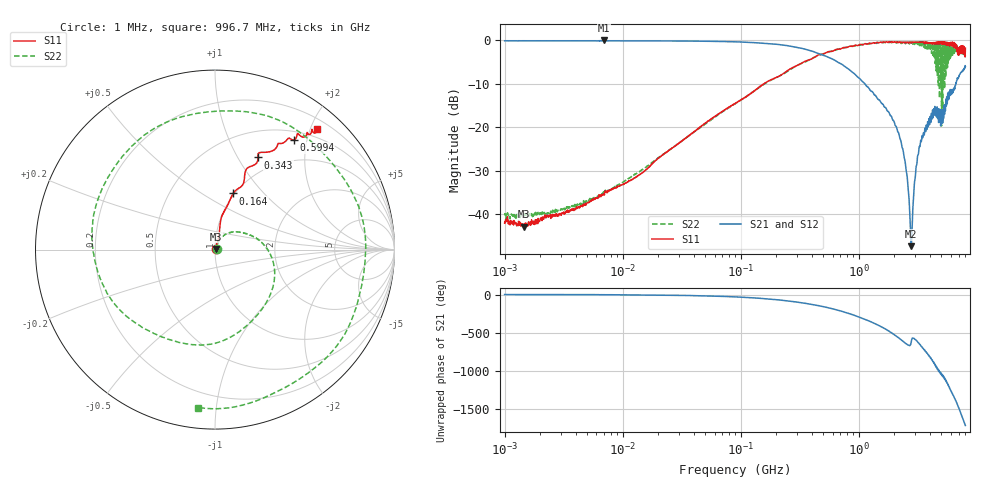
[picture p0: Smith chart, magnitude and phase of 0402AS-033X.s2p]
!s-Parameter Generated by FASTRON Sdn. Bhd.
!FASTRON P/N : 0402AS-033X
!Keysight Technologies: E5071C_MY46733604_B.14.02
!Date: Mon Dec 01 10:34:32 2025
!Version  :Rev00  Mon Dec 01 10:34:32 2025
!Data & Calibration Information:
!Freq  S11:SOLT2(ON)  S21:SOLT2(ON)  S12:SOLT2(ON)  S22:SOLT2(ON)
!PortZ  Port1:50+j0  Port2:50+j0
!When reading reference impedance value at option line is always used.
! Remarks : This data is being provided solely for informational purposes.
# Hz S dB R 50
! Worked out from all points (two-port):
!   1601 points, 1 MHz to 8 GHz, reference 50 ohm
!   highest |S21| = 0.00 dB at 6.912 MHz (marker M1); lowest = -47.4 dB at 2.78 GHz (marker M2)
!   |S21| within 3 dB of the highest: start of sweep to 452.6 MHz
!   lowest |S11| = -42.9 dB at 1.45 MHz (marker M3), VSWR 1.01, Z = 50.6 + j0.327 ohm
!   |S11| at or under -10 dB: start of sweep to 156.6 MHz
!   |S22| runs from -41.2 to -0.2 dB; largest |S21 - S12| = 0.018
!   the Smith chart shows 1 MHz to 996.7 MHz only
!   S11 on the Smith chart (normalised r, x): 1 MHz: 1.01, +0.01; 164 MHz: 0.98, +0.69; 343 MHz: 0.81, +1.22; 599.4 MHz: 0.63, +1.78; 996.7 MHz: 0.35, +2.10
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1000000  -42.10 19.6  -0.08 -0.4  -0.08 -0.4  -40.20 17.9
1450094  -42.90 26.8  -0.06 -0.5  -0.09 -0.6  -40.40 11.9
4479405  -38.10 51.7  -0.08 -1.6  -0.08 -1.6  -37.60 46.2
6911657  -35.40 53.6  0.00 -2.9  -0.12 -2.2  -34.70 49.7
2.00676e7  -27.10 71.5  -0.10 -7.1  -0.12 -7.0  -27.00 66.0
8.994653e7  -14.50 78.6  -0.32 -31.0  -0.33 -30.9  -14.60 29.4
1.639593e8  -9.66 72.1  -0.69 -55.5  -0.70 -55.4  -9.79 -9.5
3.429554e8  -4.94 65.0  -1.93 -112.0  -1.93 -112.0  -5.10 -113.0
4.006501e8  -4.23 62.0  -2.44 -130.0  -2.43 -130.0  -4.13 -145.0
5.99384e8  -2.47 54.3  -4.29 173.0  -4.29 173.0  -2.39 111.0
9.966533e8  -1.11 49.9  -8.57 68.4  -8.58 68.2  -1.06 -96.0
1.341815e9  -0.55 56.1  -12.40 -14.3  -12.40 -14.4  -0.66 91.1
1.550632e9  -0.46 61.6  -14.40 -61.1  -14.40 -61.2  -0.43 -8.1
1.7949e9  -0.32 67.7  -16.50 -117.0  -16.50 -117.0  -0.51 -127.0
2.061212e9  -0.45 73.4  -19.70 -179.0  -19.80 -179.0  -0.38 104.0
2.252141e9  -0.53 76.2  -22.90 137.0  -22.90 137.0  -0.39 10.2
2.472225e9  -0.48 81.2  -28.00 86.8  -27.90 86.8  -0.73 -101.0
2.780342e9  -0.39 90.4  -47.40 97.2  -47.40 98.5  -0.82 108.0
3.183204e9  -0.38 100.0  -26.30 91.6  -26.30 91.1  -0.76 -90.9
3.548043e9  -0.39 111.0  -21.30 3.3  -21.30 3.0  -1.55 81.5
3.933151e9  -0.65 117.0  -18.00 -81.5  -18.00 -82.0  -1.92 -91.3
8e9  -1.79 -110.0  -5.99 89.3  -6.02 88.8  -3.63 124.0
